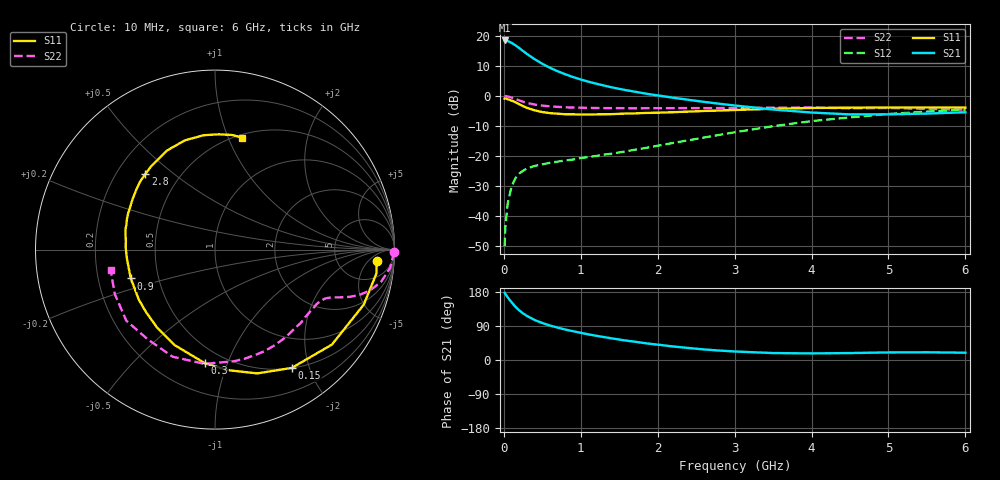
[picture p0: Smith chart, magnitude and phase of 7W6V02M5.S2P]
! Infineon Technologies  Discrete & RF Semiconductors
! BFS17W
! Si NPN RF Bipolar Junction Transistor in SOT323
! VCE = 6 V  IC = 2.5 mA
! Common Emitter S-Parameters:  August  1999
# GHz  S  MA  R  50
!  f  S11  S21  S12  S22
! GHz  MAG  ANG  MAG  ANG  MAG  ANG  MAG  ANG
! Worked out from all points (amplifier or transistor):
!   36 points, 10 MHz to 6 GHz, reference 50 ohm
!   highest |S21| = 18.4 dB at 10 MHz (marker M1)
!   |S21| within 3 dB of that: start of sweep to 223.7 MHz
!   unconditionally stable (mu >= 1): 779.5 MHz to 2.794 GHz; 4.349 GHz to end of sweep
!   at 250 MHz: K = 0.40, MSG = 19.9 dB, |S12| = -24.8 dB
!   at 1.4 GHz: K = 1.27, MAG = 7.9 dB, |S12| = -19.2 dB
!   at 6 GHz: K = 1.07, MAG = -2.1 dB, |S12| = -4.6 dB
!   S11 on the Smith chart (normalised r, x): 10 MHz: 13, -9; 150 MHz: 0.50, -1.73; 300 MHz: 0.39, -0.84; 900 MHz: 0.35, -0.15; 2.8 GHz: 0.32, +0.40; 6 GHz: 0.53, +1.13
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0.01  0.903 -4.0  8.36 177.6  0.0032 84.3  0.9989 -0.7
0.02  0.9091 -8.4  8.349 174.2  0.0066 87.7  0.9913 -2.4
0.05  0.8838 -20.3  8.177 165.4  0.0163 80.1  0.9811 -6.0
0.1  0.8392 -39.1  7.633 152.4  0.0314 70.0  0.9416 -11.1
0.15  0.7858 -57.0  6.965 140.5  0.0429 61.1  0.8909 -14.9
0.2  0.7287 -71.2  6.249 131.0  0.0514 56.2  0.8435 -17.4
0.25  0.6755 -83.9  5.572 123.0  0.0573 51.0  0.8014 -19.1
0.3  0.6359 -95.0  4.997 116.3  0.0625 48.3  0.7693 -20.2
0.4  0.5776 -113.0  4.084 105.6  0.0688 45.0  0.7201 -21.7
0.5  0.5408 -126.7  3.426 97.6  0.0733 43.9  0.6913 -22.8
0.6  0.5187 -137.7  2.932 91.0  0.0776 44.2  0.6718 -23.9
0.7  0.5078 -146.8  2.574 85.4  0.0812 45.0  0.6591 -25.3
0.9  0.496 -161.1  2.06 75.9  0.088 47.7  0.6413 -28.5
1.1  0.4925 -172.5  1.729 67.6  0.097 51.1  0.6342 -32.3
1.4  0.4988 174.6  1.394 57.2  0.1101 56.0  0.6289 -38.6
1.6  0.5115 166.9  1.241 51.0  0.1215 59.2  0.6251 -43.3
2.2  0.5379 148.8  0.937 35.7  0.1657 66.3  0.6281 -58.5
2.8  0.5727 132.7  0.743 24.9  0.2256 68.2  0.63 -75.1
3.5  0.6133 115.9  0.596 18.3  0.315 65.3  0.6393 -95.2
4.5  0.6402 95.8  0.494 18.3  0.4405 53.5  0.6247 -127.0
5.5  0.6457 81.5  0.51 20.4  0.5499 40.3  0.6107 -156.2
6  0.6417 76.2  0.537 19.2  0.5918 33.8  0.5924 -169.2
